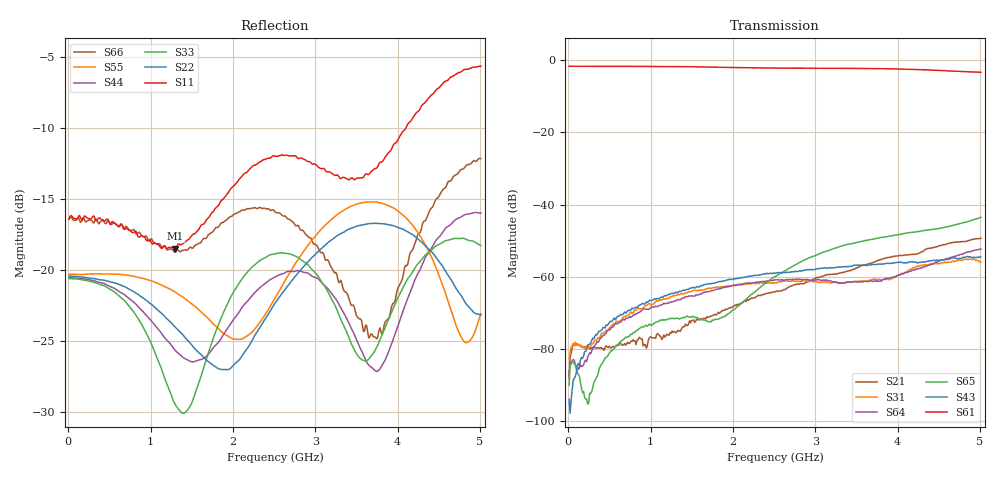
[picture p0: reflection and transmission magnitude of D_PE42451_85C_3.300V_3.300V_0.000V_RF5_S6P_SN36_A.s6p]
! Device ID: PE42451
! Serial: 36
! Insertion: A
! Temp: 85C
! VDD: 3.300
! Control_Hi: 100.000
! Control_Lo: 0.000
! Logic State: RF5
! Port 1: RFC
! Port 2: RF1
! Port 3: RF2
! Port 4: RF3
! Port 5: RF4
! Port 6: RF5
! V1 = 3.30
! V2 = 0.00
! V3 = 3.30
! V4 = 0.00
! IDD: 1.793400e-05
#  Hz  S  RI  R  50
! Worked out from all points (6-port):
!   401 points, 10 MHz to 5.01 GHz, reference 50 ohm
!   strongest paths, dB at 10 MHz, 1.26 GHz, 2.51 GHz, 3.76 GHz, 5.01 GHz:
!     S61: -1.6, -1.7, -2.1, -2.3, -3.3
!     S43: -94.0, -64.5, -59.1, -56.6, -54.5
!     S65: -90.1, -71.6, -60.0, -49.3, -43.6
!     S64: -87.3, -67.0, -60.8, -61.3, -52.4
!     S31: -83.0, -65.5, -61.7, -60.9, -56.0
!     S21: -88.1, -75.1, -64.2, -55.5, -49.3
!   lowest |S11| = -18.5 dB at 1.298 GHz (marker M1), VSWR 1.27, Z = 54.8 - j11.6 ohm
!   |S11| at or under -10 dB: start of sweep to 4.098 GHz
